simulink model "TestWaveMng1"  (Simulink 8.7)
settings: Solver=ode1  StartTime=0.0  StopTime=2  FixedStep=Tstep  RelTol=1e-3
InitFcn:
  | TestWaveMng.TestWaveMng_init();
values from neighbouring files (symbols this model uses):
  Tstep = 0.00005    (= 5e-05)    [TestWaveMng_init.m]    (also in TestOrthOscObjO_init.m = 0.0005)
libraries: lib_WaveMng x5

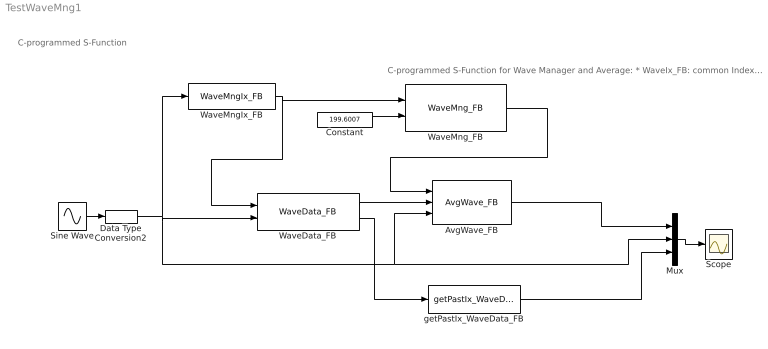
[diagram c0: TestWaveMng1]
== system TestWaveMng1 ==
  note: C-programmed S-Function
  note: C-programmed S-Function for Wave Manager and Average: * WaveIx_FB: common Index for one Buffer size. * WaveMng_FB: common manager for one average period but maybe more as one signal for averaging. * WaveData_FB; Buffer for data, for one signal value, but maybe for more as one average * AvgWave_FB: average for one signal and period. The connections ..._FB are references (ObjectOriented). The connections step... are only used to determine the calculation order.
  AvgWave_FB : lib_WaveMng/AvgWave_FB
  Constant : Constant  Value=199.6007  OutDataTypeStr=single
  Data Type Conversion2 : DataTypeConversion  OutDataTypeStr=single
  Mux : Mux  Inputs=3
  Scope : Scope
  Sine Wave : Sin  Amplitude=4  Frequency=10.02*pi  SampleTime=Tstep
  WaveData_FB : lib_WaveMng/WaveData_FB
  WaveMngIx_FB : lib_WaveMng/WaveMngIx_FB
  WaveMng_FB : lib_WaveMng/WaveMng_FB
  getPastIx_WaveData_FB : lib_WaveMng/getPastIx_WaveData_FB  ixPast=25
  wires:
  WaveMng_FB/1 -> AvgWave_FB/1
  Constant/1 -> WaveMng_FB/2
  Mux/1 -> Scope/1
  AvgWave_FB/1 -> Mux/1
  Sine Wave/1 -> Data Type Conversion2/1
  WaveMngIx_FB/1 -> WaveMng_FB/1, WaveData_FB/1
  Data Type Conversion2/1 -> WaveData_FB/2, AvgWave_FB/3, Mux/2, WaveMngIx_FB/1
  getPastIx_WaveData_FB/1 -> Mux/3
  WaveData_FB/1 -> AvgWave_FB/2
  WaveData_FB/2 -> getPastIx_WaveData_FB/1
